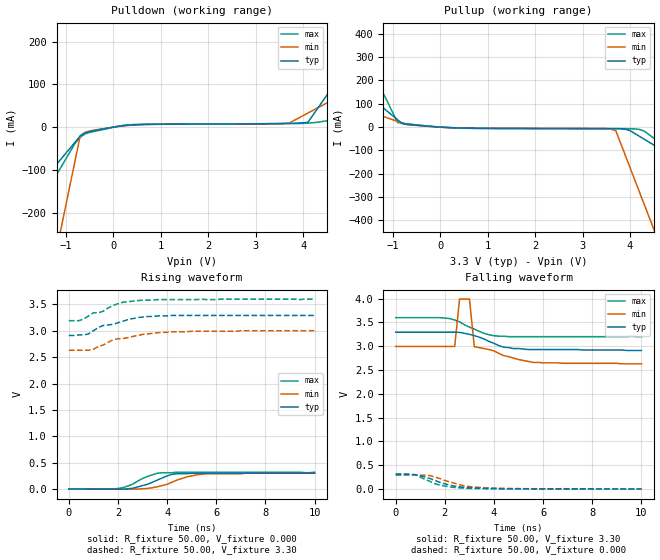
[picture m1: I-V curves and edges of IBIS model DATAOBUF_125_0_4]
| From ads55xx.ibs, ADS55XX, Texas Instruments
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|   Model DATAOBUF_125_0_4
[Model]   DATAOBUF_125_0_4
Model_type   Output
Polarity   Non-Inverting
Vmeas =   1.65V
C_comp   3.00pF   3.00pF   3.00pF
[Temperature Range]   50.00   0.10k   -20.00
[Voltage Range]   3.30V   3.00V   3.60V
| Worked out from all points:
|   slope of the pulldown table from 0 to 0.495 V, typ, clamps not added: 84.9 ohm
|   slope of the pullup table from 0 to 0.495 V, typ, clamps not added: 107 ohm
|   rising waveform, R_fixture 50.00, V_fixture 0.000: 20-80 % time 995ps typ, 1.14ns min, 866ps max; typ from 0 V to 0.3 V
|   rising waveform, R_fixture 50.00, V_fixture 3.30: 20-80 % time 1.49ns typ, 1.73ns min, 1.28ns max; typ from 2.91 V to 3.29 V
|   falling waveform, R_fixture 50.00, V_fixture 3.30: 20-80 % time 1.14ns typ, 1.32ns min, 1ns max; typ from 3.29 V to 2.91 V
|   falling waveform, R_fixture 50.00, V_fixture 0.000: 20-80 % time 1.14ns typ, 1.2ns min, 995ps max; typ from 0.3 V to 0.002 V
[Pulldown]
| voltage   I(typ)   I(min)   I(max)
-3.3V     -365.6mA   -1.417A    -506.6mA
-2.3V     -233mA     -879.5mA   -318.5mA
-1.9V     -180mA     -664.6mA   -243.2mA
-1.5V     -126.9mA   -449.7mA   -167.9mA
-1V       -60.64mA   -181.1mA   -73.79mA
-700mV    -20.86mA   -19.96mA   -23.63mA
-500mV    -10.33mA   -8.85mA    -12.35mA
400mV     5.26mA     4.7mA      5.92mA
3.7V      8.55mA     9.22mA     8.45mA
4.1V      11.37mA    32.98mA    9.43mA
5.5V      233.3mA    116.1mA    31.39mA
6.6V      407.6mA    181.5mA    49.65mA
[Pullup]
| voltage   I(typ)   I(min)   I(max)
-3.3V     436.1mA    192.3mA    1.014A
-1.9V     200mA      94.43mA    433.9mA
-900mV    31.44mA    24.53mA    19.64mA
-800mV    14.58mA    17.54mA    16.82mA
300mV     -2.94mA    -2.71mA    -3.59mA
3.6V      -6.25mA    -8.75mA    -6.53mA
3.7V      -6.37mA    -15.33mA   -6.57mA
4V        -14.93mA   -173.5mA   -6.92mA
4.2V      -39.53mA   -278.9mA   -10.01mA
4.3V      -51.83mA   -331.6mA   -16.95mA
4.5V      -76.43mA   -437mA     -47.33mA
6.6V      -334.7mA   -1.544A    -366.3mA
[Ramp]
| variable   typ   min   max
dV/dt_r   0.18/0.94n   0.18/1.14n   0.19/0.84n
dV/dt_f   0.23/1.16n   0.22/1.28n   0.24/1.01n
R_load = 50.00
[Rising Waveform]
R_fixture = 50.00
V_fixture = 0.000
V_fixture_min = 0.000
V_fixture_max = 0.000
| time   V(typ)   V(min)   V(max)
0s        17.86nV    21.45nV    37.32nV
2ns       -2.04mV    -690uV     10.17mV
2.6ns     15.91mV    -1.96mV    93.86mV
3.2ns     90.3mV     12.04mV    240mV
3.6ns     170mV      42.79mV    300mV
3.8ns     210mV      64.81mV    310mV
4.2ns     280mV      130mV      310mV
4.8ns     290mV      230mV      320mV
5.6ns     300mV      290mV      320mV
10ns      300mV      300mV      320mV
[Rising Waveform]
R_fixture = 50.00
V_fixture = 3.30
V_fixture_min = 3.00
V_fixture_max = 3.60
| time   V(typ)   V(min)   V(max)
0s        2.91V      2.63V      3.19V
400ps     2.92V      2.63V      3.19V
800ps     2.94V      2.63V      3.28V
1ns       3V         2.65V      3.34V
1.4ns     3.1V       2.73V      3.37V
1.8ns     3.12V      2.83V      3.48V
2.2ns     3.18V      2.85V      3.54V
3ns       3.26V      2.93V      3.58V
5ns       3.29V      2.99V      3.59V
10ns      3.29V      3V         3.6V
[Falling Waveform]
R_fixture = 50.00
V_fixture = 3.30
V_fixture_min = 3.00
V_fixture_max = 3.60
| time   V(typ)   V(min)   V(max)
0s        3.295V     2.995V     3.6V
1.8ns     3.295V     2.995V     3.6V
2.4ns     3.295V     2.995V     3.55V
2.6ns     3.29V      3.99V      3.51V
3ns       3.25V      3.99V      3.4V
3.2ns     3.22V      2.99V      3.36V
3.8ns     3.1V       2.93V      3.24V
4.4ns     2.98V      2.8V       3.21V
5.6ns     2.93V      2.66V      3.2V
10ns      2.91V      2.63V      3.2V
[Falling Waveform]
R_fixture = 50.00
V_fixture = 0.000
V_fixture_min = 0.000
V_fixture_max = 0.000
| time   V(typ)   V(min)   V(max)
0s        300mV      300mV      320mV
800ps     300mV      300mV      300mV
1.4ns     220mV      280mV      160mV
1.6ns     180mV      250mV      110mV
2ns       110mV      180mV      61.8mV
2.2ns     80.22mV    150mV      45.66mV
2.8ns     34.08mV    66.25mV    16.73mV
3.6ns     14.13mV    26.48mV    8.06mV
4.4ns     7.07mV     11.88mV    5mV
10ns      1.64mV     1.97mV     1.34mV
